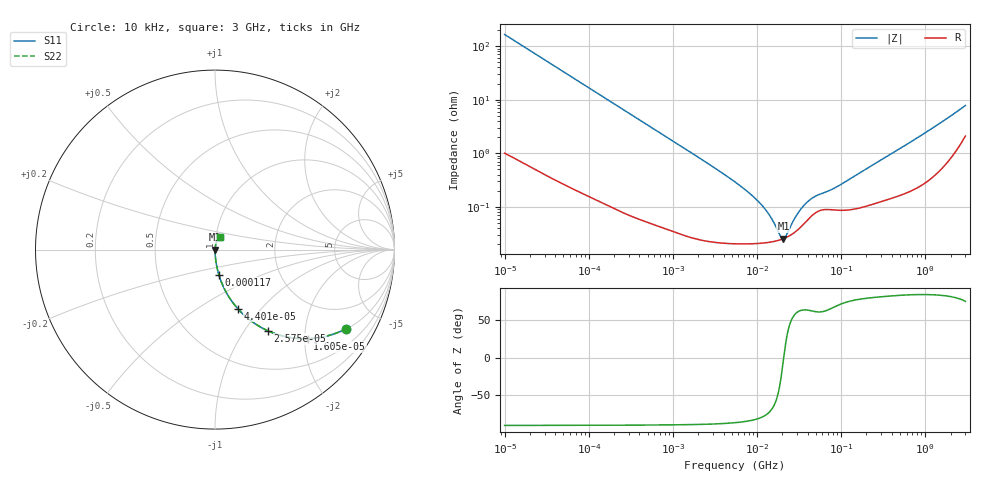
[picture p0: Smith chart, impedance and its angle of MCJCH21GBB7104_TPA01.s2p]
! MCJCH21GBB7104_TPA01  S-PARAMETER MODEL  ( Standard Model )
! Model Generated by TAIYO YUDEN Corporation (http://www.ty-top.com)
! Version 1.0
! TAIYO YUDEN Control No. 220601
! Copyright(c) 2015 TAIYO YUDEN CO.,LTD. All Rights Reserved.
! Product Description (link to TY-COMPAS)
! https://ds.yuden.co.jp/TYCOMPAS/or/detail?pn=MCJCH21GBB7104KTPA01&u=M
! Products Name : Multilayer Ceramic Capacitors
! Characteristics :
!  Capacitance : 0.1 [uF] , Rated Voltage : 100 [V] , TCC : X7R
!  Case Size : 2.0 x 1.25 / 0.079 x 0.049 [mm/inch] , Thickness : 1.25 / 0.049 [mm/inch]
!  (Conditions: Temperature = 25 [degC] , DC Bias Voltage = 0 [V])
! External Node Assignments :
!  1  o---| |---o  2
! GND o---------o GND
! Frequency Range : 10kHz  -  3GHz  [ 401 STEP ]
# MHZ S RI R 50
! Freq[MHz].  S11 Real  S11 Imag  S21 Real  S21 Imag  S12 Real  S12 Imag  S22 Real  S22 Imag
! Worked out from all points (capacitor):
!   401 points, 10 kHz to 3 GHz, reference 50 ohm
!   read as one part in series: C = 96.1 nF near 10.65 kHz
!   lowest |Z| = 25.4 mohm at 20.59 MHz (marker M1)
!   series resonance near 20.77 MHz, so ESL is about 610 pH
!   S11 on the Smith chart (normalised r, x): 10 kHz: 1.02, -3.31; 16.05 kHz: 1.01, -2.07; 25.75 kHz: 1.01, -1.29; 44.01 kHz: 1.01, -0.76; 117 kHz: 1.00, -0.29; 3 GHz: 1.04, +0.15
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0.01  0.7312 -0.4403  0.2688 0.4403  0.2688 0.4403  0.7312 -0.4403
0.016047  0.5162 -0.4965  0.4838 0.4965  0.4838 0.4965  0.5162 -0.4965
0.02575  0.2952 -0.4526  0.7048 0.4526  0.7048 0.4526  0.2952 -0.4526
0.044011  0.1271 -0.3293  0.8729 0.3293  0.8729 0.3293  0.1271 -0.3293
0.082683  0.0408 -0.1934  0.9592 0.1934  0.9592 0.1934  0.0408 -0.1934
0.11696  0.0214 -0.1398  0.9786 0.1398  0.9786 0.1398  0.0214 -0.1398
0.249268  0.0053 -0.067  0.9947 0.067  0.9947 0.067  0.0053 -0.067
0.683653  0.00104 -0.0247  0.999 0.0247  0.999 0.0247  0.00104 -0.0247
5.477226  0.000212 -0.0029  0.9998 0.0029  0.9998 0.0029  0.000212 -0.0029
8.516475  0.000206 -0.00167  0.9998 0.00167  0.9998 0.00167  0.000206 -0.00167
11.67315  0.000211 -0.00101  0.9998 0.00101  0.9998 0.00101  0.000211 -0.00101
14.55585  0.00022 -0.000603  0.9998 0.000603  0.9998 0.000603  0.00022 -0.000603
18.73182  0.000241 -0.000173  0.9998 0.000173  0.9998 0.000173  0.000241 -0.000173
20.5901  0.000253 -1.46e-05  0.9997 1.46e-05  0.9997 1.46e-05  0.000253 -1.46e-05
22.63272  0.00027 0.000144  0.9997 -0.000144  0.9997 -0.000144  0.00027 0.000144
27.34599  0.000323 0.000466  0.9997 -0.000466  0.9997 -0.000466  0.000323 0.000466
32.0153  0.000398 0.000739  0.9996 -0.000739  0.9996 -0.000739  0.000398 0.000739
37.4819  0.000511 0.001  0.9995 -0.001  0.9995 -0.001  0.000511 0.001
45.28751  0.00069 0.00128  0.9993 -0.00128  0.9993 -0.00128  0.00069 0.00128
90.61918  0.000868 0.00224  0.9991 -0.00224  0.9991 -0.00224  0.000868 0.00224
374.4521  0.00148 0.00915  0.9985 -0.00915  0.9985 -0.00915  0.00148 0.00915
3000  0.0258 0.0716  0.9742 -0.0716  0.9742 -0.0716  0.0258 0.0716
